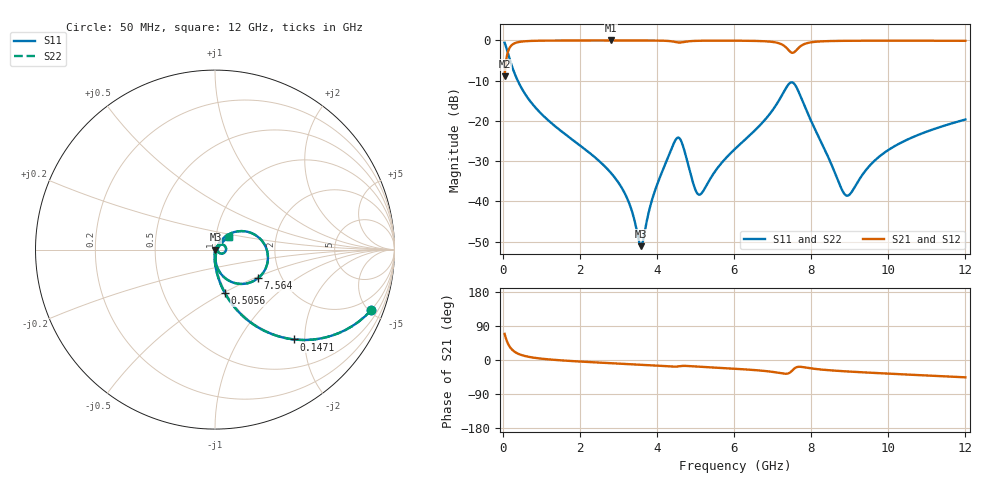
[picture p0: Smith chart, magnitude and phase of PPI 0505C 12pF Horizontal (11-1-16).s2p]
# MHz S MA R 50
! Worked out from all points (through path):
!   1601 points, 50 MHz to 12 GHz, reference 50 ohm
!   highest |S21| = -0.02 dB at 2.799 GHz (marker M1); lowest = -9.0 dB at 50 MHz (marker M2)
!   group delay of S21, straight-line fit = 12.8 ps
!   lowest |S11| = -51.1 dB at 3.59 GHz (marker M3), VSWR 1.01, Z = 50.3 - j0.0734 ohm
!   |S11| at or under -10 dB: 389.7 MHz to end of sweep
!   |S22| runs from -51.1 to -0.6 dB; largest |S21 - S12| = 0
!   S11 on the Smith chart (normalised r, x): 50 MHz: 0.99, -5.20; 147.1 MHz: 0.99, -1.77; 505.6 MHz: 0.99, -0.51; 7.564 GHz: 1.52, -0.53; 12 GHz: 1.16, +0.16
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50  0.9343 -21.1  0.3564 68.9  0.3564 68.9  0.9343 -21.1
147.0938  0.6647 -48.8  0.7468 41.1  0.7468 41.1  0.6647 -48.8
281.5312  0.4203 -66.0  0.9068 23.9  0.9068 23.9  0.4203 -66.0
505.5938  0.2474 -77.2  0.9681 12.6  0.9681 12.6  0.2474 -77.2
1050.812  0.1161 -86.4  0.9921 3.0  0.9921 3.0  0.1161 -86.4
2044.156  0.04795 -92.6  0.9973 -4.3  0.9973 -4.3  0.04795 -92.6
2798.5  0.02284 -93.8  0.9978 -8.3  0.9978 -8.3  0.02284 -93.8
3239.156  0.01061 -88.9  0.9976 -10.6  0.9976 -10.6  0.01061 -88.9
3590.188  0.002777 -15.3  0.997 -12.3  0.997 -12.3  0.002777 -15.3
4038.312  0.01783 55.8  0.9937 -14.8  0.9937 -14.8  0.01783 55.8
4531.25  0.06157 10.1  0.9446 -17.2  0.9446 -17.2  0.06157 10.1
4650.75  0.05297 -20.7  0.9469 -15.7  0.9469 -15.7  0.05297 -20.7
4964.438  0.01544 -25.2  0.9844 -16.9  0.9844 -16.9  0.01544 -25.2
5091.406  0.01212 4.1  0.9884 -17.7  0.9884 -17.7  0.01212 4.1
6025  0.0448 57.6  0.9914 -23.1  0.9914 -23.1  0.0448 57.6
7227.469  0.2022 29.8  0.8968 -35.1  0.8968 -35.1  0.2022 29.8
7436.594  0.2922 -2.7  0.7382 -34.0  0.7382 -34.0  0.2922 -2.7
7563.562  0.2882 -33.4  0.715 -22.6  0.715 -22.6  0.2882 -33.4
8019.156  0.09501 -83.4  0.95 -22.4  0.95 -22.4  0.09501 -83.4
8915.406  0.0118 -25.3  0.9877 -30.1  0.9877 -30.1  0.0118 -25.3
10013.31  0.04385 44.3  0.9911 -36.0  0.9911 -36.0  0.04385 44.3
12000  0.104 40.8  0.9876 -45.7  0.9876 -45.7  0.104 40.8
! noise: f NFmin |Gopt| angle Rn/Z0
50  0.000408  0.8742  1.578  0.0006995
1372  0.004094  0.6815  5.106  0.002483
2701  0.006955  0.6408  9.465  0.003634
4031  0.01529  0.7424  13.81  0.01174
5360  0.02043  0.7451  18.31  0.01571
6682  0.03166  0.7913  22.62  0.03011
8012  0.06158  0.8673  27.18  0.09427
9341  0.0289  0.7028  31.35  0.01771
1.067e+04  0.02637  0.6453  35.27  0.01285
1.2e+04  0.02704  0.622  39.07  0.01195
